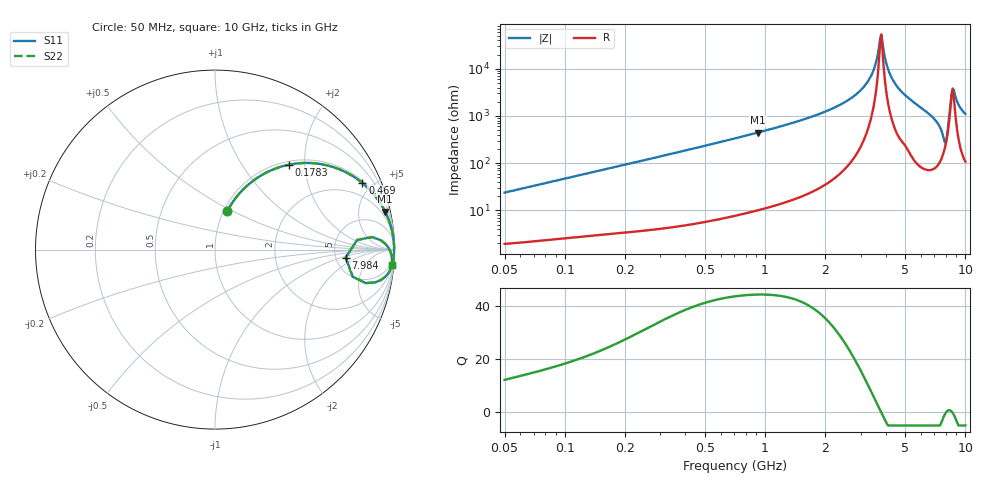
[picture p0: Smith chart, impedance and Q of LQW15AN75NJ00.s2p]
!Murata Part Number: LQW15AN75NJ00
!These Parameters are Measured in Series Mode Connection
!  o--[Z]--o
!Port1  Port2
!  o-------o
!Freq. Start=50[MHz] Stop=10[GHz], 401[Steps]
# Hz S RI R 50
!Freq.(Hz)	S 11(Real)	S 11(Imag)	S 21(Real)	S 21(Imag)	S 12(Real)	S 12(Imag)	S 22(Real)	S 22(Imag)
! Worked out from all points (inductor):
!   401 points, 50 MHz to 10 GHz, reference 50 ohm
!   read as one part in series: L = 75.2 nH near 51.34 MHz
!   highest Q = 44.3 at 921.6 MHz (marker M1), where L = 77 nH
!   self-resonance near 3.752 GHz
!   S11 on the Smith chart (normalised r, x): 50 MHz: 1.04, +0.47; 178.3 MHz: 1.06, +1.66; 469 MHz: 1.11, +4.37; 7.984 GHz: 6.18, -1.17; 10 GHz: 3, -22
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5e7  0.0695 0.2166  0.9305 -0.2166  0.9305 -0.2166  0.0695 0.2166
1.214486e8  0.2544 0.4118  0.7456 -0.4118  0.7456 -0.4118  0.2544 0.4118
1.78327e8  0.4111 0.4729  0.5889 -0.4729  0.5889 -0.4729  0.4111 0.4729
2.949953e8  0.6479 0.4631  0.3521 -0.4631  0.3521 -0.4631  0.6479 0.4631
4.689809e8  0.821 0.3712  0.179 -0.3712  0.179 -0.3712  0.821 0.3712
7.071068e8  0.9129 0.2708  0.0871 -0.2708  0.0871 -0.2708  0.9129 0.2708
9.215873e8  0.9478 0.2114  0.0522 -0.2114  0.0522 -0.2114  0.9478 0.2114
1.717543e9  0.987 0.1013  0.013 -0.1013  0.013 -0.1013  0.987 0.1013
2.423676e9  0.995 0.0545  0.00497 -0.0545  0.00497 -0.0545  0.995 0.0545
3.035766e9  0.9975 0.0269  0.00253 -0.0269  0.00253 -0.0269  0.9975 0.0269
3.420121e9  0.9981 0.0125  0.00195 -0.0125  0.00195 -0.0125  0.9981 0.0125
3.558764e9  0.9981 0.00775  0.00186 -0.00775  0.00186 -0.00775  0.9981 0.00775
3.703027e9  0.9982 0.00292  0.00183 -0.00292  0.00183 -0.00292  0.9982 0.00292
3.802437e9  0.9982 -0.000324  0.00185 0.000324  0.00185 0.000324  0.9982 -0.000324
4.171863e9  0.9979 -0.0119  0.00213 0.0119  0.00213 0.0119  0.9979 -0.0119
4.826234e9  0.9962 -0.0311  0.00379 0.0311  0.00379 0.0311  0.9962 -0.0311
7.086521e9  0.9737 -0.1179  0.0263 0.1179  0.0263 0.1179  0.9737 -0.1179
7.672705e9  0.8922 -0.183  0.1078 0.183  0.1078 0.183  0.8922 -0.183
7.983737e9  0.7284 -0.0441  0.2716 0.0441  0.2716 0.0441  0.7284 -0.0441
8.307378e9  0.9258 0.0513  0.0742 -0.0513  0.0742 -0.0513  0.9258 0.0513
8.644138e9  0.9755 -0.00692  0.0245 0.00692  0.0245 0.00692  0.9755 -0.00692
1e10  0.9835 -0.0876  0.0165 0.0876  0.0165 0.0876  0.9835 -0.0876
